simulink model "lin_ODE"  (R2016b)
settings: Solver=VariableStepAuto  StartTime=0.0  StopTime=10  RelTol=1e-3

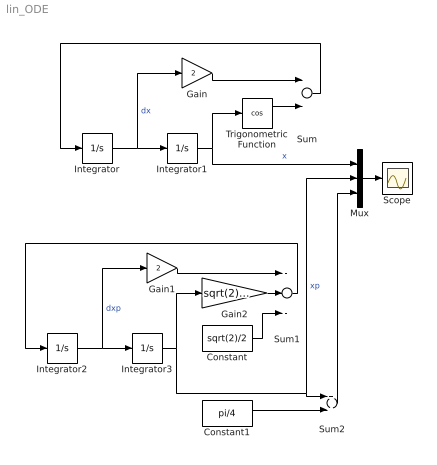
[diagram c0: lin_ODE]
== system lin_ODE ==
  Constant : Constant  Value=sqrt(2)/2
  Constant1 : Constant  Value=pi/4
  Gain : Gain  Gain=2
  Gain1 : Gain  Gain=2
  Gain2 : Gain  Gain=sqrt(2)/2
  Integrator : Integrator
  Integrator1 : Integrator  InitialCondition=pi/4
  Integrator2 : Integrator
  Integrator3 : Integrator
  Mux : Mux  Inputs=3
  Scope : Scope
  Sum : Sum  Inputs=--
  Sum1 : Sum  Inputs=-+-
  Sum2 : Sum
  Trigonometric Function : Trigonometry  Operator=cos
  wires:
  Integrator/1 -> Gain/1, Integrator1/1  "dx"
  Integrator1/1 -> Mux/1, Trigonometric Function/1  "x"
  Trigonometric Function/1 -> Sum/2
  Sum/1 -> Integrator/1
  Gain/1 -> Sum/1
  Integrator2/1 -> Gain1/1, Integrator3/1  "dxp"
  Integrator3/1 -> Mux/2, Sum2/1, Gain2/1  "xp"
  Gain2/1 -> Sum1/2
  Sum1/1 -> Integrator2/1
  Gain1/1 -> Sum1/1
  Constant/1 -> Sum1/3
  Mux/1 -> Scope/1
  Constant1/1 -> Sum2/2
  Sum2/1 -> Mux/3
